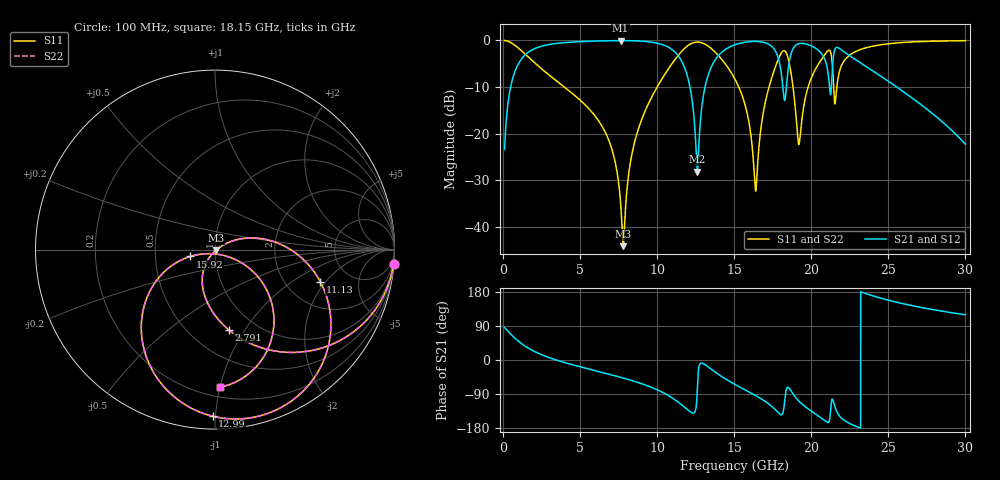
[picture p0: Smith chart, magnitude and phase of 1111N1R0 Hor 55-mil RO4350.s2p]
# GHz S MA R 50
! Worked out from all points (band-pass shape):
!   3201 points, 100 MHz to 30 GHz, reference 50 ohm
!   highest |S21| = -0.06 dB at 7.622 GHz (marker M1); lowest = -28.1 dB at 12.6 GHz (marker M2)
!   |S21| within 3 dB of the highest: 1.446 GHz to 11.31 GHz (9.862 GHz wide, 155 % of centre); 14.03 GHz to 17.78 GHz (3.752 GHz wide, 23.6 % of centre)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
!   lowest |S11| = -44.1 dB at 7.799 GHz (marker M3), VSWR 1.01, Z = 50.4 - j0.483 ohm
!   |S11| at or under -10 dB: 3.975 GHz to 9.996 GHz (6.021 GHz wide, 86.2 % of centre); 15.3 GHz to 17.26 GHz (1.963 GHz wide, 12.1 % of centre); 18.82 GHz to 19.79 GHz (977.1 MHz wide, 5.06 % of centre)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
!   |S22| runs from -44.1 to 0.0 dB; largest |S21 - S12| = 0
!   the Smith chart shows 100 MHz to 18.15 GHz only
!   S11 on the Smith chart (normalised r, x): 100 MHz: 1, -25; 2.791 GHz: 0.75, -0.85; 11.13 GHz: 3.07, -1.77; 12.99 GHz: 0.07, -0.98; 15.92 GHz: 0.76, -0.06; 18.15 GHz: 0.27, -1.00
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0.1  0.9977 -4.5  0.06785 85.5  0.06785 85.5  0.9977 -4.5
0.8755312  0.8583 -36.4  0.5123 53.6  0.5123 53.6  0.8583 -36.4
2.791  0.4521 -80.4  0.8895 9.3  0.8895 9.3  0.4521 -80.4
5.089563  0.222 -107.9  0.971 -18.8  0.971 -18.8  0.222 -107.9
7.621719  0.01855 -116.9  0.993 -45.6  0.993 -45.6  0.01855 -116.9
7.79925  0.00625 -50.0  0.9929 -47.6  0.9929 -47.6  0.00625 -50.0
8.518719  0.07923 28.1  0.9882 -56.3  0.9882 -56.3  0.07923 28.1
10.06978  0.3319 7.6  0.9274 -79.8  0.9274 -79.8  0.3319 7.6
11.12562  0.614 -17.0  0.7575 -104.2  0.7575 -104.2  0.614 -17.0
12.60194  0.9594 -74.1  0.0393 -77.0  0.0393 -77.0  0.9594 -74.1
12.99437  0.9284 -90.8  0.2532 -9.5  0.2532 -9.5  0.9284 -90.8
15.05  0.3836 -151.0  0.8988 -64.5  0.8988 -64.5  0.3836 -151.0
15.91897  0.143 -164.5  0.9662 -83.4  0.9662 -83.4  0.143 -164.5
16.41419  0.02531 -79.4  0.9738 -94.4  0.9738 -94.4  0.02531 -79.4
18.15213  0.7676 -88.1  0.3204 -139.9  0.3204 -139.9  0.7676 -88.1
18.56325  0.5773 -134.9  0.5777 -74.5  0.5777 -74.5  0.5773 -134.9
19.18928  0.07674 -101.4  0.9217 -108.3  0.9217 -108.3  0.07674 -101.4
20.03956  0.4096 -52.1  0.8669 -136.0  0.8669 -136.0  0.4096 -52.1
21.31966  0.6541 -123.9  0.3537 -106.9  0.3537 -106.9  0.6541 -123.9
21.97372  0.5432 -69.3  0.7867 -153.9  0.7867 -153.9  0.5432 -69.3
25.01978  0.9204 -113.7  0.363 157.6  0.363 157.6  0.9204 -113.7
30  0.9914 -152.4  0.07725 119.4  0.07725 119.4  0.9914 -152.4
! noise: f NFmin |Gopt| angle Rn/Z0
0.1  0.002997  0.947  2.195  0.01268
3.417  0.01318  0.589  24.82  0.005614
6.743  0.02467  0.5749  42.34  0.009249
10.06  0.05281  0.6903  58.99  0.02541
13.39  0.1825  0.8719  79.4  0.1823
16.7  0.08971  0.7031  95.1  0.02798
20.03  0.1299  0.7503  110.7  0.03533
23.35  0.1353  0.7373  123.3  0.02508
26.67  0.2261  0.8342  137.8  0.03947
30  0.5631  0.932  154.3  0.09336
